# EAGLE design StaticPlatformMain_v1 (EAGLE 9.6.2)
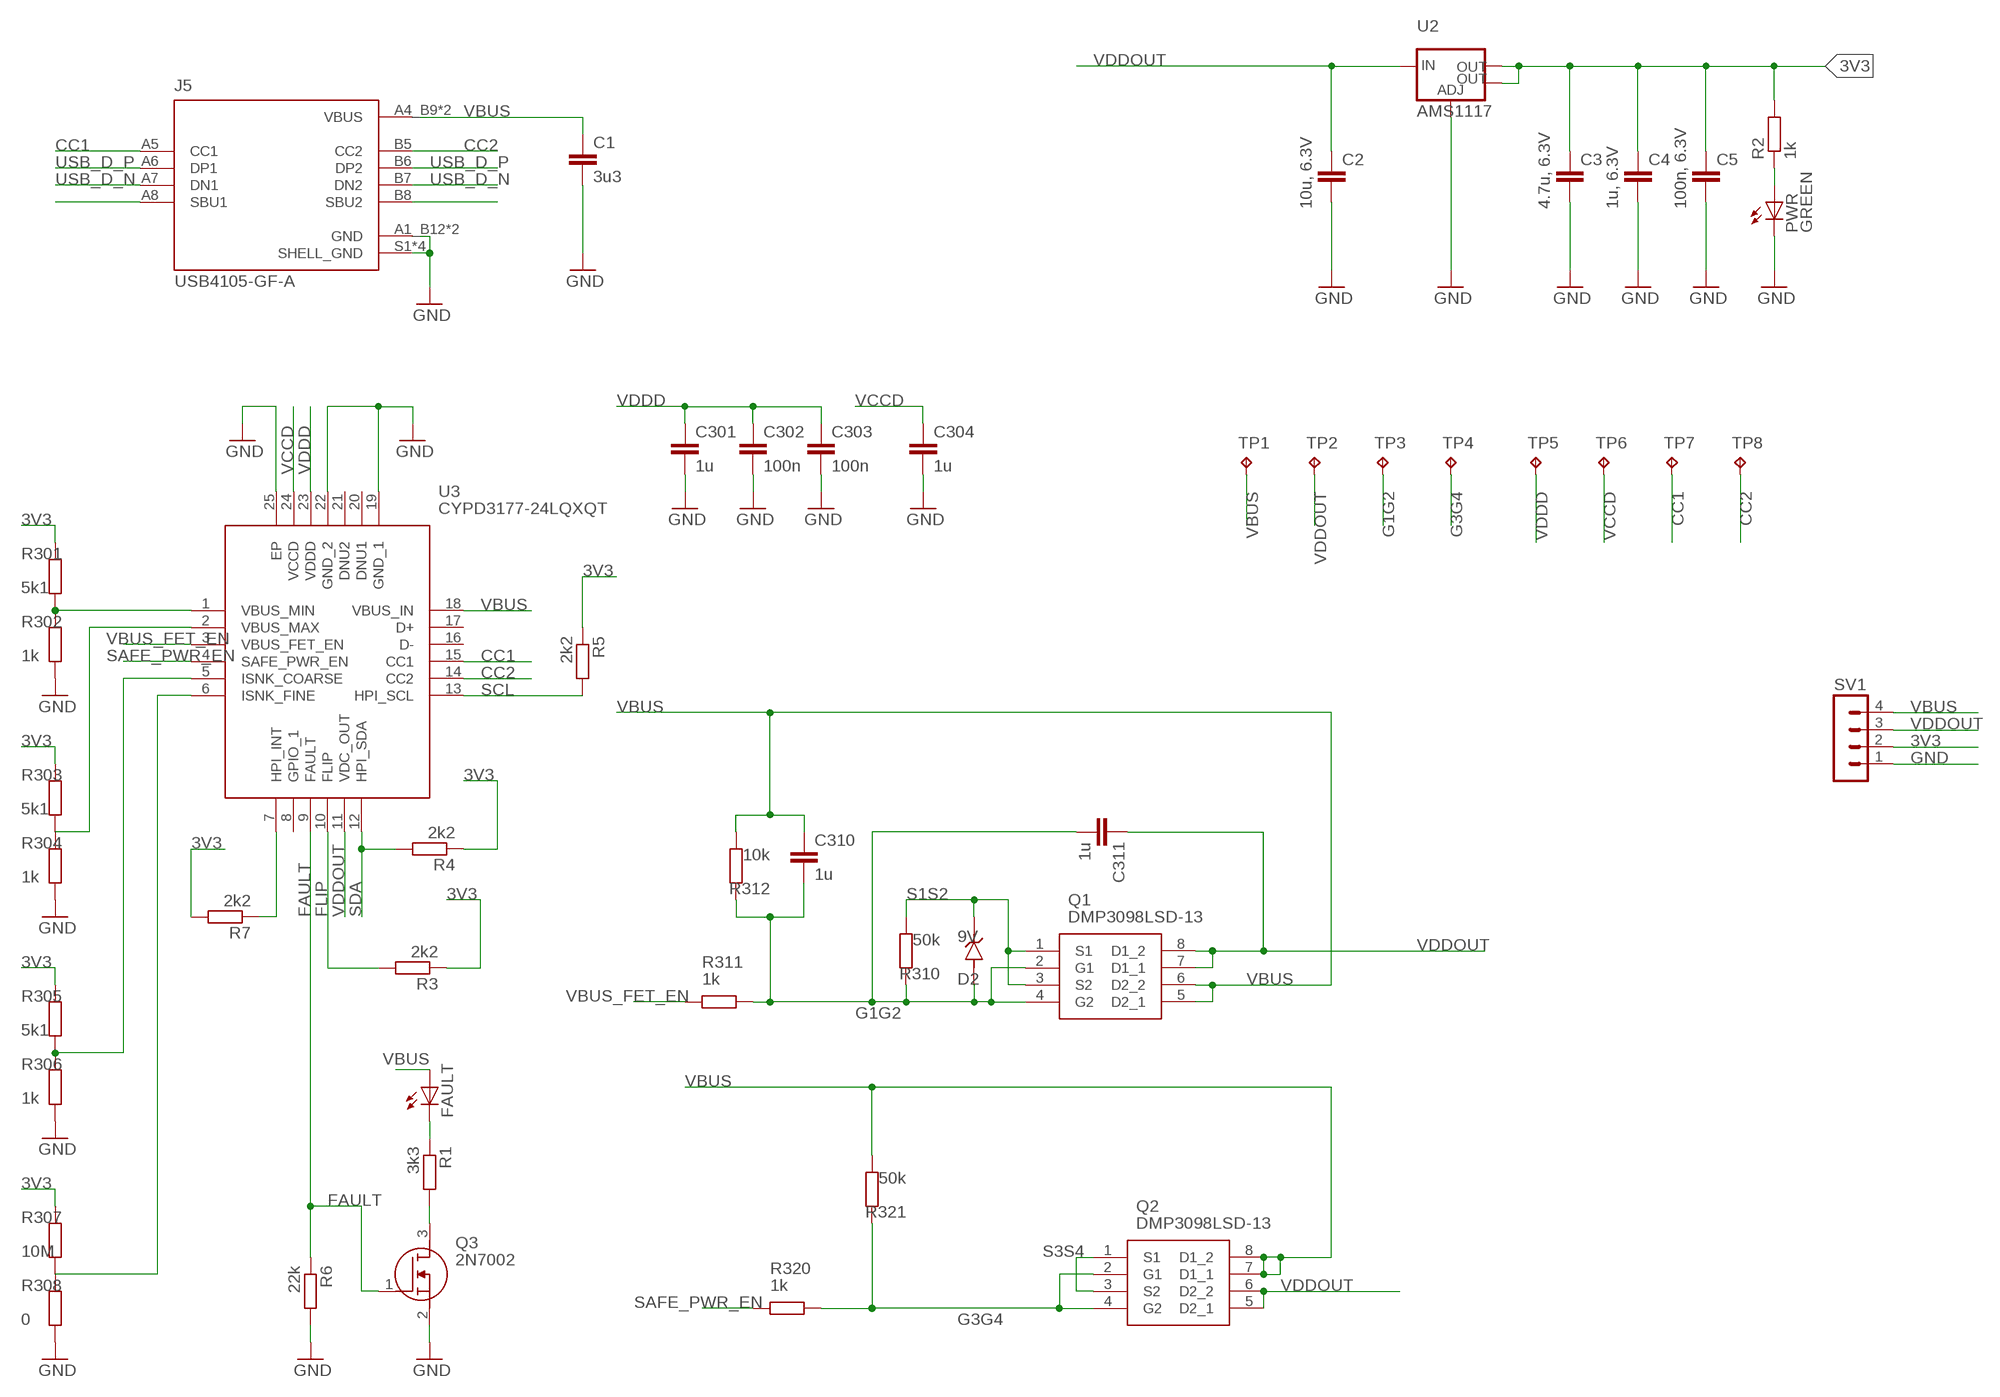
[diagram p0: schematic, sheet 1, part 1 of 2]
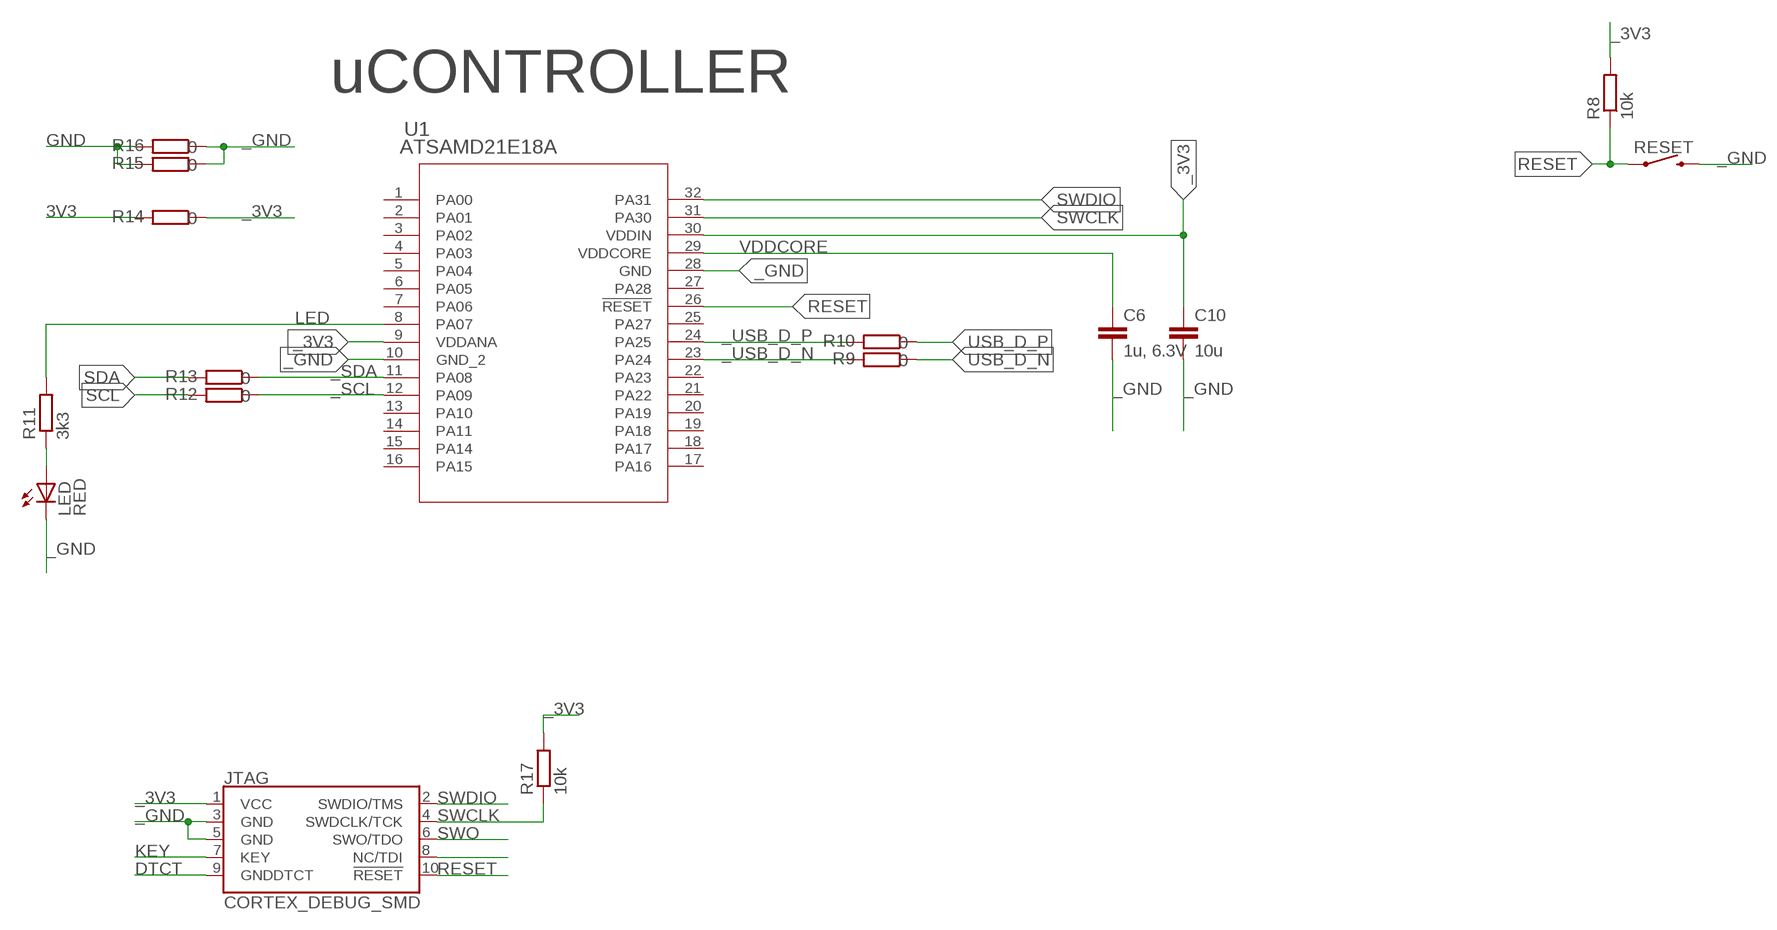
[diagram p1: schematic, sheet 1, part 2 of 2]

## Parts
C1  3u3  C-EUC0805K  [C0805K]
C2  10u, 6.3V  C-EUC0805K  [C0805K]
C3  4.7u, 6.3V  C-EUC0805K  [C0805K]
C4  1u, 6.3V  C-EUC0805K  [C0805K]
C5  100n, 6.3V  C-EUC0805K  [C0805K]
C6  1u, 6.3V  C-EUC0805  [C0805]
C10  10u  C-EUC0805  [C0805]
C301  1u  C-EUC0805K  [C0805K]
C302  100n  C-EUC0805K  [C0805K]
C303  100n  C-EUC0805K  [C0805K]
C304  1u  C-EUC0805K  [C0805K]
C310  1u  C-EUC0805K  [C0805K]
C311  1u  C-EUC0805K  [C0805K]
D2  9V  BZV55C12_L0G  [DIOMELF3515N]
FAULT  GREEN  LEDCHIPLED_0805  [CHIPLED_0805]
J5  USB4105-GF-A  [GCT_USB4105-GF-A]
JTAG  CORTEX_DEBUG_SMD  [SAMTECH_FTSH-105-01]
LED  RED  LEDCHIPLED_0805  [CHIPLED_0805]
PWR  GREEN  LEDCHIPLED_0805  [CHIPLED_0805]
Q1  DMP3098LSD-13  [SOIC127P600X175-8N]
Q2  DMP3098LSD-13  [SOIC127P600X175-8N]
Q3  2N7002  [SOT96P240X120-3N]
R1  3k3  R-EU_R0805  [R0805]
R2  1k  R-EU_R0805  [R0805]
R3  2k2  R-EU_R0805  [R0805]
R4  2k2  R-EU_R0805  [R0805]
R5  2k2  R-EU_R0805  [R0805]
R6  22k  R-EU_R0805  [R0805]
R7  2k2  R-EU_R0805  [R0805]
R8  10k  R-EU_R0805  [R0805]
R9  0  R-EU_R0805  [R0805]
R10  0  R-EU_R0805  [R0805]
R11  3k3  R-EU_R0805  [R0805]
R12  0  R-EU_R0805  [R0805]
R13  0  R-EU_R0805  [R0805]
R14  0  R-EU_R0805  [R0805]
R15  0  R-EU_R0805  [R0805]
R16  0  R-EU_R0805  [R0805]
R17  10k  R-EU_R0805  [R0805]
R301  5k1  R-EU_R0805  [R0805]
R302  1k  R-EU_R0805  [R0805]
R303  5k1  R-EU_R0805  [R0805]
R304  1k  R-EU_R0805  [R0805]
R305  5k1  R-EU_R0805  [R0805]
R306  1k  R-EU_R0805  [R0805]
R307  10M  R-EU_R0805  [R0805]
R308  0  R-EU_R0805  [R0805]
R310  50k  R-EU_R0805  [R0805]
R311  1k  R-EU_R0805  [R0805]
R312  10k  R-EU_R0805  [R0805]
R320  1k  R-EU_R0805  [R0805]
R321  50k  R-EU_R0805  [R0805]
RESET  MOMENTARY-SWITCH-SPST-SMD-6.0X3.5MM  [TACTILE_SWITCH_SMD_6.0X3.5MM]
SV1  MA04-1  [MA04-1]
TP1  TPTP18R  [TP18R]
TP2  TPTP18R  [TP18R]
TP3  TPTP18R  [TP18R]
TP4  TPTP18R  [TP18R]
TP5  TPTP18R  [TP18R]
TP6  TPTP18R  [TP18R]
TP7  TPTP18R  [TP18R]
TP8  TPTP18R  [TP18R]
U1  ATSAMD21E18A  ATSAMD21E18A-AUTQFP32_MC_MCH-M  [TQFP32_MC_MCH-M]
U2  AMS1117  V_REG_LM1117SOT223  [SOT223]
U3  CYPD3177-24LQXQT  [QFN50P400X400X60-25N]

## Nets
3V3: C3.1 C4.1 C5.1 R2.2 R3.1 R4.1 R5.1 R7.2 R14.2 R301.2 R303.2 R305.2 R307.2 SV1.2 U2.2(OUT) U2.4(OUT)
_3V3: C10.1 JTAG.1(VCC) R8.2 R14.1 R17.2 U1.9(VDDANA) U1.30(VDDIN)
_GND: C6.2 C10.2 JTAG.3(GND) JTAG.5(GND) LED.C R15.1 R16.1 RESET.2 U1.10(GND_2) U1.28(GND)
_SCL: R12.1 U1.12(PA09)
_SDA: R13.1 U1.11(PA08)
_USB_D_N [usbpair]: R9.2 U1.23(PA24)
_USB_D_P [usbpair]: R10.2 U1.24(PA25)
CC1: J5.A5(CC1) TP7.TP U3.15(CC1)
CC2: J5.B5(CC2) TP8.TP U3.14(CC2)
DTCT: JTAG.9(GNDDTCT)
FAULT: Q3.1(G) R6.1 U3.9(FAULT)
FLIP: R3.2 U3.10(FLIP)
G1G2: C310.2 C311.2 D2.A Q1.2(G1) Q1.4(G2) R310.2 R311.1 R312.2 TP3.TP
G3G4: Q2.2(G1) Q2.4(G2) R320.1 R321.2 TP4.TP
GND: C1.2 C2.2 C3.2 C4.2 C5.2 C301.2 C302.2 C303.2 C304.2 J5.A1_B12(GND) J5.B1_A12(GND) J5.S1(SHELL_GND) J5.S2(SHELL_GND) J5.S3(SHELL_GND) J5.S4(SHELL_GND) PWR.C Q3.2(S) R6.2 R15.2 R16.2 R302.1 R304.1 R306.1 R308.1 SV1.1 U2.1(ADJ) U3.19(GND_1) U3.22(GND_2) U3.25(EP)
KEY: JTAG.7(KEY)
LED: R11.2 U1.8(PA07)
LED_GP: LED.A R11.1
LED_PWR: PWR.A R2.1
N$1: FAULT.C R1.1
N$2: R7.1 U3.7(HPI_INT)
N$3: R301.1 R302.2 U3.1(VBUS_MIN)
N$4: R303.1 R304.2 U3.2(VBUS_MAX)
N$5: R305.1 R306.2 U3.5(ISNK_COARSE)
N$7: Q3.3(D) R1.2
N$9: J5.A8(SBU1)
N$10: R307.1 R308.2 U3.6(ISNK_FINE)
N$19: J5.B8(SBU2)
N$24: JTAG.8(NC/TDI)
RESET: JTAG.10(!RESET) R8.1 RESET.1 U1.26(!RESET)
S1S2: D2.C(K) Q1.1(S1) Q1.3(S2) R310.1
S3S4: Q2.1(S1) Q2.3(S2)
SAFE_PWR_EN: R320.2 U3.4(SAFE_PWR_EN)
SCL: R5.2 R12.2 U3.13(HPI_SCL)
SDA: R4.2 R13.2 U3.12(HPI_SDA)
SWCLK: JTAG.4(SWDCLK/TCK) R17.1 U1.31(PA30)
SWDIO: JTAG.2(SWDIO/TMS) U1.32(PA31)
SWO: JTAG.6(SWO/TDO)
USB_D_N [usbpair]: J5.A7(DN1) J5.B7(DN2) R9.1
USB_D_P [usbpair]: J5.A6(DP1) J5.B6(DP2) R10.1
VBUS: C1.1 C310.1 FAULT.A J5.A4_B9(VBUS) J5.B4_A9(VBUS) Q1.5(D2_1) Q1.6(D2_2) Q2.7(D1_1) Q2.8(D1_2) R312.1 R321.1 SV1.4 TP1.TP U3.18(VBUS_IN)
VBUS_FET_EN: R311.2 U3.3(VBUS_FET_EN)
VCCD: C304.1 TP6.TP U3.24(VCCD)
VDDCORE: C6.1 U1.29(VDDCORE)
VDDD: C301.1 C302.1 C303.1 TP5.TP U3.23(VDDD)
VDDOUT: C2.1 C311.1 Q1.7(D1_1) Q1.8(D1_2) Q2.5(D2_1) Q2.6(D2_2) SV1.3 TP2.TP U2.3(IN) U3.11(VDC_OUT)
Unconnected: U1.1(PA00) U1.2(PA01) U1.3(PA02) U1.4(PA03) U1.5(PA04) U1.6(PA05) U1.7(PA06) U1.13(PA10) U1.14(PA11) U1.15(PA14) U1.16(PA15) U1.17(PA16) U1.18(PA17) U1.19(PA18) U1.20(PA19) U1.21(PA22) U1.22(PA23) U1.25(PA27) U1.27(PA28) U3.8(GPIO_1) U3.16(D-) U3.17(D+) U3.20(DNU1) U3.21(DNU2)

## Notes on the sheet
- uCONTROLLER

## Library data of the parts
C1-C6 C10 C301-C304 C310 C311 = rcl:C-EU: CAPACITOR, European symbol; SPICEPREFIX: C
D2 = BZV55C12_L0G:BZV55C12_L0G: Check availability; AVAILABILITY: In Stock; CHECK_PRICES: https://www.snapeda.com/parts/BZV55C12%20L0G/Taiwan+Semiconductor/view-part/?ref=eda; DESCRIPTION: MMELF, 500mW, 5%, Small Signal Zener Diode; MF: Taiwan Semiconductor Corporation; MP: BZV55C12 L0G; PACKAGE: MINI MELF-2-2 Taiwan Semiconductor; PRICE: None; PURCHASE-URL: https://www.snapeda.com/api/url_track_click_mouser/?unipart_id=6304637&manufacturer=Taiwan Semiconductor Corporation&part_name=BZV55C12 L0G&search_term=None; SNAPEDA_LINK: https://www.snapeda.com/parts/BZV55C12%20L0G/Taiwan+Semiconductor/view-part/?ref=snap
FAULT LED PWR = adafruit:LED: LED
J5 = USB4105-GF-A:USB4105-GF-A: USB-C (USB TYPE-C) USB 2.0 Receptacle Connector 24 (16+8 Dummy) Position Surface Mount, Right Angle; Through Hole Check availability; AVAILABILITY: In Stock; DESCRIPTION: USB-C (USB TYPE-C) USB 2.0 Receptacle Connector 24 (16+8 Dummy) Position Surface Mount, Right Angle; Through Hole; MF: GCT; MP: USB4105-GF-A; PACKAGE: None; PRICE: None; PURCHASE-URL: https://pricing.snapeda.com/search?q=USB4105-GF-A&ref=eda
JTAG = SparkFun-Connectors:CORTEX_DEBUG: Cortex Debug Connector - 10 pin Supports JTAG debug, Serial Wire debug, and Serial Wire Viewer. PTH and SMD connector options available. General Connector Information Products: PTH Connector -via Digi-Key SparkFun PSoc SparkFun T
Q1 Q2 = DMP3098LSD-13:DMP3098LSD-13: MOSFET PMOS-DUAL Source: Datasheet; DESCRIPTION: MOSFET PMOS-DUAL; HEIGHT: 1.75mm; MANUFACTURER_NAME: Diodes Inc.; MANUFACTURER_PART_NUMBER: DMP3098LSD-13; MOUSER_PART_NUMBER: 621-DMP3098LSD-13; MOUSER_PRICE-STOCK: https://www.mouser.co.uk/ProductDetail/Diodes-Incorporated/DMP3098LSD-13?qs=oUsD4qhOtFxafARAi3NzqQ%3D%3D
Q3 = 2N7002:2N7002: N-channel MOSFET,2N7002 0.115A 60V Source: Datasheet; DESCRIPTION: N-channel MOSFET,2N7002 0.115A 60V; HEIGHT: 1.2mm; MANUFACTURER_NAME: onsemi; MANUFACTURER_PART_NUMBER: 2N7002; MOUSER_PART_NUMBER: 512-2N7002; MOUSER_PRICE-STOCK: https://www.mouser.co.uk/ProductDetail/onsemi-Fairchild/2N7002?qs=0dwsXDNhqlz66WJJhrTFjQ%3D%3D
R1-R17 R301-R308 R310-R312 R320 R321 = rcl:R-EU_: RESISTOR, European symbol; SPICEPREFIX: R
RESET = SparkFun-Switches:MOMENTARY-SWITCH-SPST: Momentary Switch (Pushbutton) - SPST; PROD_ID: SWCH-14278; SF_SKU: COM-08229
SV1 = con-lstb_round_pads:MA04-1: PIN HEADER; OC_FARNELL: unknown; OC_NEWARK: unknown
TP1-TP8 = testpad:TP: Test pad
U1 = SAMD21E18:ATSAMD21E18A-AU; COPYRIGHT: Copyright (C) 2022 Ultra Librarian. All rights reserved.; MANUFACTURER_PART_NUMBER: ATSAMD21E18A-AU; MFR_NAME: Microchip
U2 = SparkFun-IC-Power:V_REG_LM1117: Voltage Regulator LM1117 Standard adjustable voltage regulator but in SMD form. Spark Fun Electronics SKU : COM-00595; PROD_ID: VREG-08170
U3 = CYPD3177-24LQXQT:CYPD3177-24LQXQT: USB Type-C DFP Port Controller USB 1.1 3.3V/5V T/R 24-Pin QFN EP Source: Datasheet; DESCRIPTION: USB Type-C DFP Port Controller USB 1.1 3.3V/5V T/R 24-Pin QFN EP; HEIGHT: 0.6mm; MANUFACTURER_NAME: Cypress Semiconductor; MANUFACTURER_PART_NUMBER: CYPD3177-24LQXQT; MOUSER_PART_NUMBER: 727-CYPD3177-24LQXQT; MOUSER_PRICE-STOCK: https://www.mouser.co.uk/ProductDetail/Cypress-Semiconductor/CYPD3177-24LQXQT?qs=PzGy0jfpSMvUfBLYWBYBLA%3D%3D

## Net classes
1 usbpair: width 0.25 mm, clearance 0.2 mm

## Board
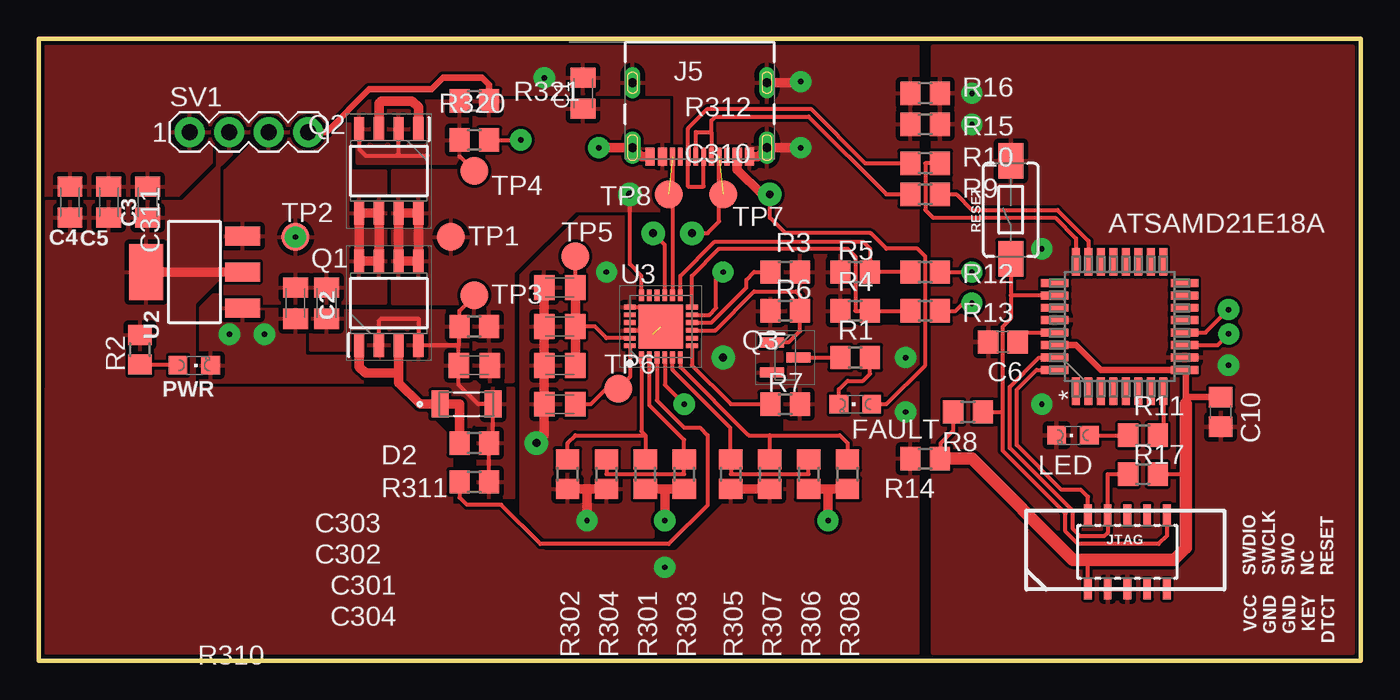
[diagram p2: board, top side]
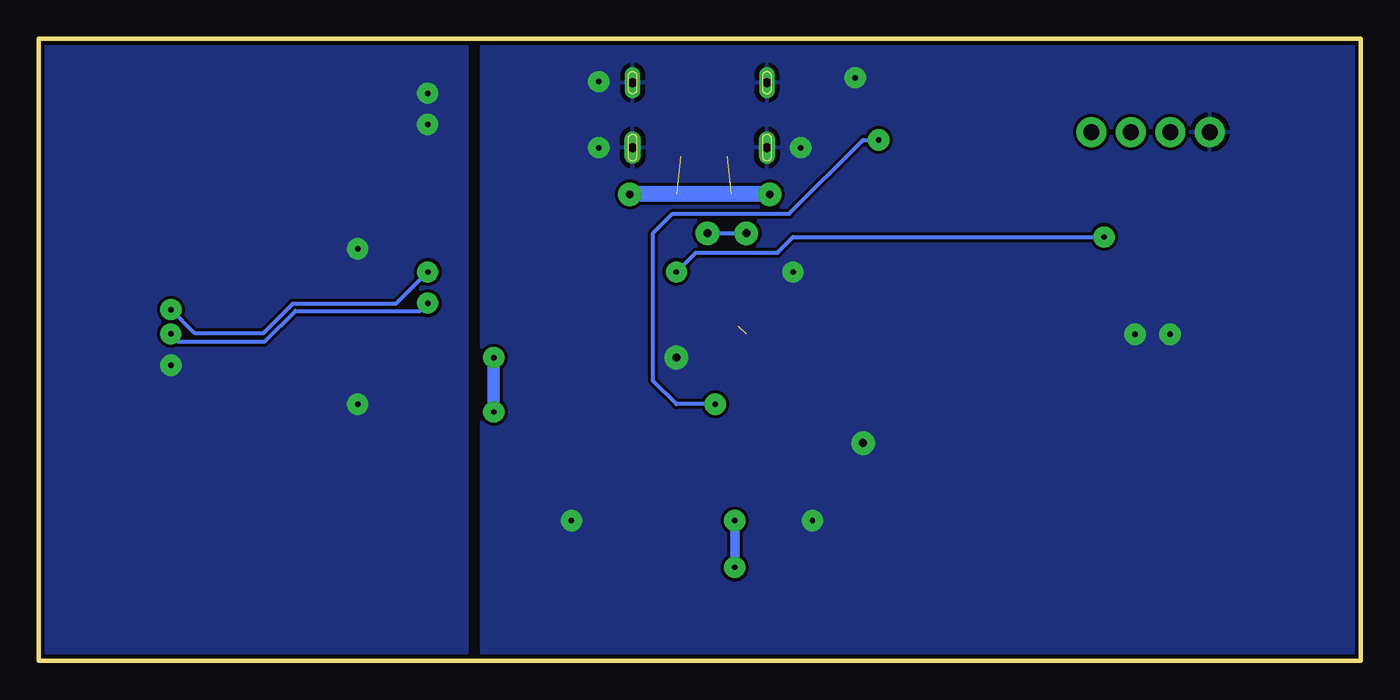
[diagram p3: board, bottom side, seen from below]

Size 85 x 40 mm. Coordinates in mm from the lower left corner, seen from the top.
Outline: 0,40 85,40 85,0 0,0 0,40
Copper layers (1*16): Top 0.035mm / dielectric 1.5mm / Bottom 0.035mm
Design rules "default *": minimum track width 0.25mm, minimum drill 0.35mm, track to track 0.2mm, track to pad 0.2mm, pad to pad 0.2mm, via to via 0.2mm, smd to smd 0.2mm, copper to edge 0.2mm, drill to drill 0.2mm, minimum pad ring 8mil, minimum via ring 1mm, stop-mask expansion 4mil, vias tented up to drill 0mil, thermal gap 12mil
tRestrict: 2 lines

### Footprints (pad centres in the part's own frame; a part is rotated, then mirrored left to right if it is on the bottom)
C0805K = smd 1.3 x 1.6: 1 -1,0; 2 1,0
C0805 = smd 1.3 x 1.5: 1 -0.95,0; 2 0.95,0
DIOMELF3515N = smd 1.11 x 1.73: A 1.705,0; C -1.705,0
CHIPLED_0805 = smd 1.2 x 1.2: A 0,-1.05; C 0,1.05
GCT_USB4105-GF-A = smd 0.6 x 1.15: A1_B12 -3.2,4.755; A4_B9 -2.4,4.755; B1_A12 3.2,4.755; B4_A9 2.4,4.755 | smd 0.3 x 1.15: A5 -1.25,4.755; A6 -0.25,4.755; A7 0.25,4.755; A8 1.25,4.755; B5 1.75,4.755; B6 0.75,4.755; B7 -0.75,4.755; B8 -1.75,4.755 | drill 0.6 pad 1.05 long: S1 -4.32,4.18; S4 4.32,4.18 | drill 0.6 pad 1 long: S2 -4.32,0; S3 4.32,0
SAMTECH_FTSH-105-01 = smd 0.508 x 1.27: 1 -2.54,-2.413; 2 -2.54,2.413; 3 -1.27,-2.413; 4 -1.27,2.413; 5 0,-2.413; 6 0,2.413; 7 1.27,-2.413; 8 1.27,2.413; 9 2.54,-2.413; 10 2.54,2.413
SOIC127P600X175-8N = smd 1.5 x 0.65: 1 -2.7,1.905; 2 -2.7,0.635; 3 -2.7,-0.635; 4 -2.7,-1.905; 5 2.7,-1.905; 6 2.7,-0.635; 7 2.7,0.635; 8 2.7,1.905
SOT96P240X120-3N = smd 1.55 x 0.65: 1 -0.85,0.96; 2 -0.85,-0.96; 3 0.85,0
R0805 = smd 1.3 x 1.5: 1 -0.95,0; 2 0.95,0
TACTILE_SWITCH_SMD_6.0X3.5MM = smd 2.3 x 1.6: 1 -3.15,0; 2 3.15,0
MA04-1 = drill 1.016 pad 1.93: 1 -3.81,0; 2 -1.27,0; 3 1.27,0; 4 3.81,0
TP18R = smd 1.8 x 1.8: TP 0,0
TQFP32_MC_MCH-M = smd 1.762 x 0.507: 1 -4.169,2.8; 2 -4.169,2; 3 -4.169,1.2; 4 -4.169,0.4; 5 -4.169,-0.4; 6 -4.169,-1.2; 7 -4.169,-2; 8 -4.169,-2.8; 17 4.169,-2.8; 18 4.169,-2; 19 4.169,-1.2; 20 4.169,-0.4; 21 4.169,0.4; 22 4.169,1.2; 23 4.169,2; 24 4.169,2.8 | smd 0.507 x 1.762: 9 -2.8,-4.169; 10 -2,-4.169; 11 -1.2,-4.169; 12 -0.4,-4.169; 13 0.4,-4.169; 14 1.2,-4.169; 15 2,-4.169; 16 2.8,-4.169; 25 2.8,4.169; 26 2,4.169; 27 1.2,4.169; 28 0.4,4.169; 29 -0.4,4.169; 30 -1.2,4.169; 31 -2,4.169; 32 -2.8,4.169
SOT223 = smd 1.219 x 2.235: 1 -2.311,-3.099; 2 0,-3.099; 3 2.311,-3.099 | smd 3.6 x 2.2: 4 0,3.099
QFN50P400X400X60-25N = smd 0.75 x 0.3: 1 -2,1.25; 2 -2,0.75; 3 -2,0.25; 4 -2,-0.25; 5 -2,-0.75; 6 -2,-1.25; 13 2,-1.25; 14 2,-0.75; 15 2,-0.25; 16 2,0.25; 17 2,0.75; 18 2,1.25 | smd 0.3 x 0.75: 7 -1.25,-2; 8 -0.75,-2; 9 -0.25,-2; 10 0.25,-2; 11 0.75,-2; 12 1.25,-2; 19 1.25,2; 20 0.75,2; 21 0.25,2; 22 -0.25,2; 23 -0.75,2; 24 -1.25,2 | smd 2.85 x 2.85: 25 0,0

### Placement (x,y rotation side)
C1  35,36.5 90 top
C2  16.5,23 270 top
C3  7,29.5 90 top
C4  2,29.5 90 top
C5  4.5,29.5 90 top
C6  62,20.5 180 top
C10  76,16 270 top
C301  33.5,19 180 top
C302  33.5,21.5 180 top
C303  33.5,24 180 top
C304  33.5,16.5 180 top
C310  28,19 180 top
C311  18.5,23 270 top
D2  27.5,16.5 0 top
FAULT  52.5,16.5 90 top
J5  42.5,37.18 180 top
JTAG  70,7 0 top
LED  66.5,14.5 90 top
PWR  10,19 270 top
Q1  22.5,23 90 top
Q2  22.5,31.5 270 top
Q3  48,19.5 0 top
R1  52.5,19.5 180 top
R2  6.5,20 90 top
R3  48,25 180 top
R4  52.5,22.5 0 top
R5  52.5,25 0 top
R6  48,22.5 180 top
R7  48,16.5 0 top
R8  59.75,16 180 top
R9  57,30 0 top
R10  57,32 0 top
R11  71,14.5 0 top
R12  57,25 180 top
R13  57,22.5 180 top
R14  57,13 180 top
R15  57,34.5 180 top
R16  57,36.5 180 top
R17  71,12 0 top
R301  39,12 270 top
R302  34,12 90 top
R303  41.5,12 270 top
R304  36.5,12 90 top
R305  44.5,12 270 top
R306  49.5,12 90 top
R307  47,12 270 top
R308  52,12 90 top
R310  28,14 0 top
R311  28,11.5 180 top
R312  28,21.5 180 top
R320  28,33.5 0 top
R321  28,36 180 top
RESET  62.5,29 90 top
SV1  13.5,34 0 top
TP1  26.5,27.25 0 top
TP2  16.5,27.25 0 top
TP3  28,23.5 0 top
TP4  28,31.5 0 top
TP5  34.5,26 0 top
TP6  37.25,17.5 0 top
TP7  44,30 0 top
TP8  40.5,30 0 top
U1  69.5,21.5 90 top
U2  10,25 90 top
U3  40,21.5 90 top

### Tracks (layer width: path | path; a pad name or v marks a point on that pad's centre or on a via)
3V3  (via drill 0.35)
  Top 0.61: R301.2 40,11.05 | 40,11.05 R303.2 | 40,11.05 40.25,10.8 v40.25,9 | R305.2 46,11.05 R307.2 | U2.2 U2.4
  Bottom 0.61: v40.25,9 v40.25,6
  Bottom 0.813: v55.75,16 v55.75,19.5
  pour Top (rank 2): 11.5,34.5 11.5,31.75 9.25,29.5 0.5,29.5 0.5,14 10,14 10,23 14.5,27.5 14.5,34.5
  pour Top (rank 2): 0.5,17.5 23.25,17.5 26.5,14.25 26.5,10 29.5,10 32.5,7 41,7 44.5,10.5 48,10.5 48,21.5 56.5,21.5 56.5,0.5 0.5,0.5
  pour Top (rank 2): 48,27 48,21 52.5,21 52.5,27
_3V3
  Top 0.25: 73.75,18.62 U1.9 | R17.2 73.75,12 | R14.1 58,13.05 58,14 58.8,14.8 R8.2 | JTAG.1 67.46,6.46 67.5,6.5
  Top 0.406: U1.9 68.3,18.7 66.7,20.3 U1.30 | 73.75,16.5 73.75,17 | 73.75,17 73.75,18.62 | C10.1 73.8,16.95 73.75,17
  Top 0.813: R14.1 60,13 66.5,6.5 67.5,6.5 73,6.5 73.75,7.25 73.75,12 73.75,16.5
_GND  (via drill 0.35)
  other vias: 60,36.5 60,34.5 64.5,26.5 64.5,16.5 76.5,19
  pour Top (rank 4): 57.5,39.5 57.5,0.5 84.5,0.5 84.5,39.5
  pour Bottom (rank 4): 57.5,39.5 57.5,0.5 84.5,0.5 84.5,39.5
_SCL  (via drill 0.35)
  Top 0.25: R12.1 v60,25 | v76.5,22.58 75.02,21.1 U1.12
  Bottom 0.25: v60,25 62.05,22.95 68.69,22.95 70.55,21.08 75,21.08 v76.5,22.58
_SDA  (via drill 0.35)
  Top 0.25: v60,23 59.45,23 58.95,22.5 R13.1 | U1.11 75.8,20.3 v76.52,21.02
  Bottom 0.25: v60,23 60.5,22.5 68.5,22.5 70.48,20.52 76.02,20.52 v76.52,21.02
_USB_D_N
  Top 0.25: R9.2 59,30 60,29 65.5,29 67.5,27 U1.23
_USB_D_P
  Top 0.25: R10.2 57.02,32 57,31.98 57,29 57.5,28.5 65.36,28.5 66.7,27.16 U1.24
CC1  (via drill 0.5)  (1 unrouted)
  Top 0.25: U3.15 40.25,26.75 v39.5,27.5 | v42,27.5 43,27.5 43.75,28.25 J5.A5
  Bottom 0.25: v42,27.5 v39.5,27.5
CC2  (1 unrouted)
  Top 0.25: J5.B5 U3.14
FAULT
  Top 0.25: U3.9 43.5,21.25 46,23.75 48.7,23.75 48.95,23.5 R6.1 48.95,21.2 48.25,20.5 47.19,20.5 Q3.1
FLIP
  Top 0.25: U3.10 43.25,21.75 45.5,24 45.5,24.5 46,25 R3.2
G1G2
  Top 0.25: Q1.2 21.86,21.86 22,22 24.41,22 Q1.4 26.95,20.3 27,20.25 | R311.1 R310.2 29.2,14.26 D2.A 28.25,16.5 27,17.75 C310.2 27,20.25 | 27,20.25 27,21.45 R312.2 27.05,22.5 28,23.45 TP3.TP
  pour Top (rank 2): 30.5,17.5 30.5,10.5 28,10.5 28,13.5 21.5,20 17.5,20 17.5,22.5 28,22.5 28,18 28.5,17.5
G3G4
  Top 0.25: Q2.4 20.59,32.91 21,32.5 23,32.5 | 23,32.5 23.14,32.63 Q2.2 | 23,32.5 25,32.5 | TP4.TP 27.05,32.45
  pour Top (rank 2): 27.5,36 27.5,32 20.5,32 20.5,36
GND  (via drill 0.35, 0.5)  (1 unrouted)
  Top 0.25: U3.22 39.25,21.25 39.5,21 | U3.19 38.75,22.75 39,22.5
  Top 0.61: C303.2 C302.2 C301.2 C304.2 32.5,14.5 v32,14 | R302.1 35.5,11.05 | 35.5,11.05 R304.1 | 35.5,11.05 35.25,10.8 v35.25,9 | R306.1 51,11.05 | 51,11.05 R308.1 | 51,11.05 50.75,10.8 v50.75,9 | v36,33 J5.S4 38.76,32.43 J5.B1_A12 | v49,33 J5.S1 46.24,32.43 J5.A1_B12 | J5.S2 48.93,37.18 v49,37.25
  other vias: 14.5,21 12.25,21 44,19.5 36.5,25 32.5,37.5
  pour Top (rank 3): 39.5,28.5 34.5,28.5 31,25 31,9.5 32.5,8 39.5,8
  pour Top (rank 3): 48,16.5 44.5,16.5 42.5,18.5 42.5,20.5 46,24 48,24
  pour Top (rank 3): 56.5,27 0.5,27 0.5,39.5 56.5,39.5
  pour Top (rank 3): 10,23.5 10,17 21,17 21,19.5 17,23.5
  pour Bottom (rank 4): 0.5,39.5 0.5,0.5 56.5,0.5 56.5,39.5
LED
  Top 0.25: U1.8 72.3,14.85 R11.2
LED_GP
  Top 0.25: LED.A R11.1
LED_PWR
  Top 0.25: R2.1 8.9,19.05 PWR.A
N$1
  Top 0.25: FAULT.C 51.45,17.45 52,18 53,18 53.45,18.45 R1.1
N$2
  Top 0.25: R7.1 44.5,16.5 42,19 U3.7
N$3
  Top 0.25: U3.1 38.75,14.75 39,14.5 | 39,14.5 R301.1 | R302.2 34,14 34.5,14.5 39,14.5
N$4
  Top 0.25: U3.2 39.25,16.45 41.5,14.2 R303.1 41.5,12 36.5,12 R304.2
N$5
  Top 0.25: U3.5 40.75,18.7 44.48,14.97 44.48,12.97 R305.1 44.5,12 49.5,12 R306.2
N$7
  Top 0.25: Q3.3 R1.2
N$10
  Top 0.25: U3.6 41.25,18.89 45.64,14.5 47,14.5 | 47,14.5 51.5,14.5 52,14 R308.2 | R307.1 47,14.5
RESET
  Top 0.25: U1.26 62.5,23.5 | 61.99,16 61.99,13.49 66.02,9.46 66.02,8.3 66.83,7.5 72,7.5 72.54,8.04 JTAG.10 | 61.99,16 61.99,21.49 62.5,22 62.5,23.5 | RESET.1 62.5,23.5 | R8.1 61.99,16
S1S2
  Top 0.61: Q1.1 20.59,18.91 21,18.5 23.14,18.5 Q1.3 23.14,17.86 24.5,16.5 D2.C 27.05,16.5 R310.1
S3S4
  Top 0.61: Q2.3 21.86,35.87 22,36 24,36 24.41,35.59 Q2.1
SAFE_PWR_EN  (via drill 0.35)
  Top 0.25: U3.4 40.25,17.75 v41.5,16.5 | R320.2 v31,33.5
  Bottom 0.25: v41.5,16.5 44,16.5 45.5,18 45.5,27.5 44.25,28.75 36.75,28.75 32,33.5 v31,33.5
SCL
  Top 0.25: U3.13 41.25,24.75 43.45,26.95 53,26.95 53.45,26.5 R5.2 R12.2
SDA
  Top 0.25: U3.12 42,24.75 43.75,26.5 52,26.5 52.5,26 52.5,22.5 R4.2 R13.2
SWCLK
  Top 0.25: U1.31 64.33,19.5 62.44,17.62 62.44,13.68 66.5,9.62 66.5,8.46 66.96,8 68.5,8 68.73,8.23 JTAG.4 68.73,12 R17.1
SWDIO
  Top 0.25: JTAG.2 67.46,10.54 67,11 65.76,11 62.89,13.87 62.89,17.43 64.16,18.7 U1.32
USB_D_N
  Top 0.25: J5.A7 42.25,34 43.25,34 | 43.25,34 J5.B7 | 43.25,34 43.25,34.75 43.5,35 49.5,35 54.5,30 R9.1
USB_D_P
  Top 0.25: R10.1 53.14,32 49.64,35.5 43,35.5 41.75,34.25 J5.B6 41.75,30.5 42.75,30.5 J5.A6
VBUS  (via drill 0.5)
  Top 0.25: U3.18 38.75,24.75 38,25.5 v38,30 | FAULT.A 54.5,16.5 57,19 57,26 56.5,26.5 54.5,26.5 53.5,27.5 48,27.5 47,28.5 v47,30
  Top 0.406: R321.1 28.95,37.05 28.5,37.5 26,37.5 25.25,36.75 21.25,36.75 18.5,34 SV1.4
  Top 0.61: J5.B4_A9 40.1,32.1 | J5.A4_B9 44.9,31.6 46.5,30 v47,30 | Q1.6 Q2.7 Q2.8 Q1.5 Q1.6
  Bottom 1.016: v38,30 v47,30
  pour Top: 22.75,31.5 22.75,23 28,23 28,18 30.5,18 30.5,25 34.5,29 40,29 40.5,29.5 40.5,36 28,36 28,31.5
VBUS_FET_EN
  Top 0.25: U3.3 39.75,16.75 41.5,15 42.5,15 43,14.5 43,10 40.5,7.5 32.25,7.5 29.73,10.03 27.52,10.03 27.05,10.5 R311.2
VCCD
  Top 0.25: C304.1 35.5,16.5 36.5,17.5 TP6.TP 38,18.25 U3.24
VDDCORE
  Top 0.25: C6.1 63.55,21.1 U1.29
VDDD
  Top 0.25: C302.1 35.75,21.5 36.5,20.75 U3.23 | C303.1 TP5.TP
  Top 0.61: C301.1 C302.1 C303.1
VDDOUT  (via drill 0.35)
  Top 0.25: U3.11 43.11,22.25 43.55,22.69 43.55,24.55 v44,25
  Top 0.61: Q1.8 Q2.5 Q2.6 Q1.7 Q1.8
  Bottom 0.25: v44,25 42.75,26.25 37.5,26.25 36.5,27.25 TP2.TP
  other vias: 16.5,27.25
  pour Top: 22.25,31.5 22.25,23 12,23 12,31.5 15,34.5 20,34.5 20,31.5

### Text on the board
tNames: SWDIO | SWCLK | SWO | NC | RESET | VCC | GND | GND | KEY | DTCT

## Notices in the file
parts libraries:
SparkFun-IC-Power: Licensing: Creative Commons ShareAlike 4.0 International - https://creativecommons.org/licenses/by-sa/4.0
